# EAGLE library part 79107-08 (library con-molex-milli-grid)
RECEPTACAL
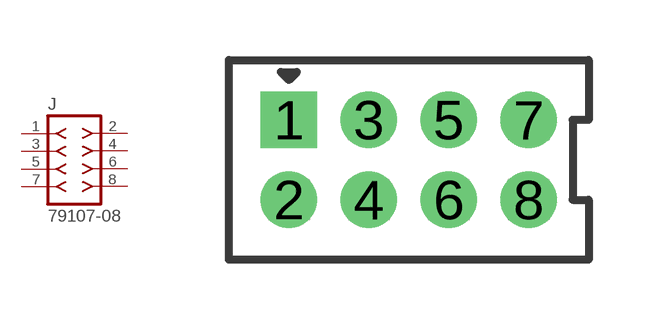
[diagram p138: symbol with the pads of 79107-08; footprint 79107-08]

Designator prefix J

## 79107-08  [79107-08]
1  1  pas
2  2  pas
3  3  pas
4  4  pas
5  5  pas
6  6  pas
7  7  pas
8  8  pas

## Footprint 79107-08 (pad centres in mm)
RECEPTACAL Dual Row, Vertical, Through-Hole
drill 0.914 square: 1 -3,1
drill 0.914: 2 -3,-1; 3 -1,1; 4 -1,-1; 5 1,1; 6 1,-1; 7 3,1; 8 3,-1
